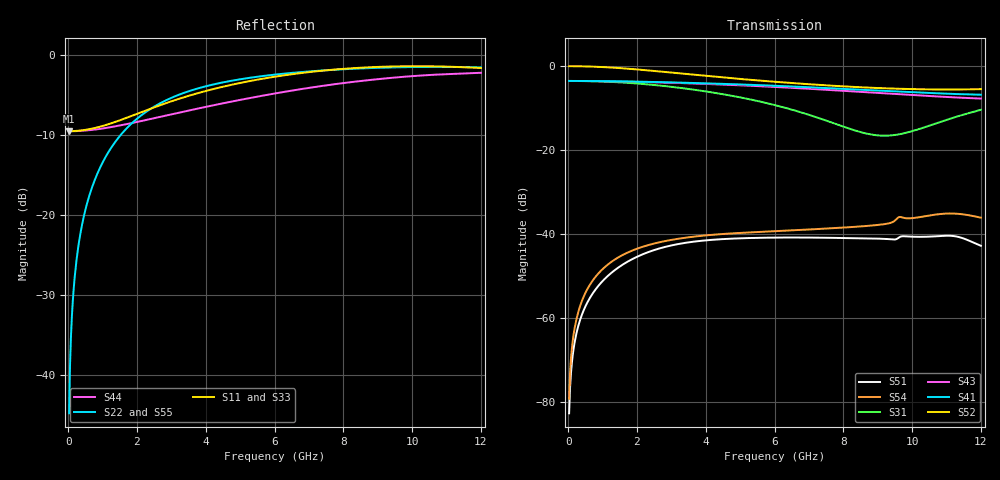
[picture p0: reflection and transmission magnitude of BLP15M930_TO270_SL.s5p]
! Touchstone file from project BLP15M930_TO270
! Exported from HFSS 2017.2.0
! Variables:
!  AirBox_H = 20mm
!  AirBox_L = 30mm
!  AirBox_W = 60mm
!  pcb_h = 502um
# GHZ S MA R 50.000000
! Terminal data exported
! Port[1] = P2_BWT2_5_Rect_T1
! Port[2] = P5_BWT3_Rect_T1
! Port[3] = P16_BWT6_Rect_T1
! Port[4] = Box3_T1
! Port[5] = Box2_T1
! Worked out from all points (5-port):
!   450 points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, 26.67 MHz to 12 GHz, reference per port
!   strongest paths, dB at 26.67 MHz, 3.013 GHz, 6.027 GHz, 9.013 GHz, 12 GHz:
!     S52: 0.0, -1.5, -3.7, -5.2, -5.5
!     S41: -3.5, -3.9, -4.7, -5.8, -6.8
!     S43: -3.5, -4.0, -5.0, -6.4, -7.7
!     S31: -3.5, -4.9, -9.3, -16.5, -10.4
!     S54: -79.3, -41.4, -39.4, -37.9, -36.1
!     S51: -82.8, -42.7, -40.9, -41.1, -42.8
!   lowest |S11| = -9.5 dB at 26.67 MHz (marker M1), VSWR 2.00
!   |S11| at or under -10 dB: nowhere
